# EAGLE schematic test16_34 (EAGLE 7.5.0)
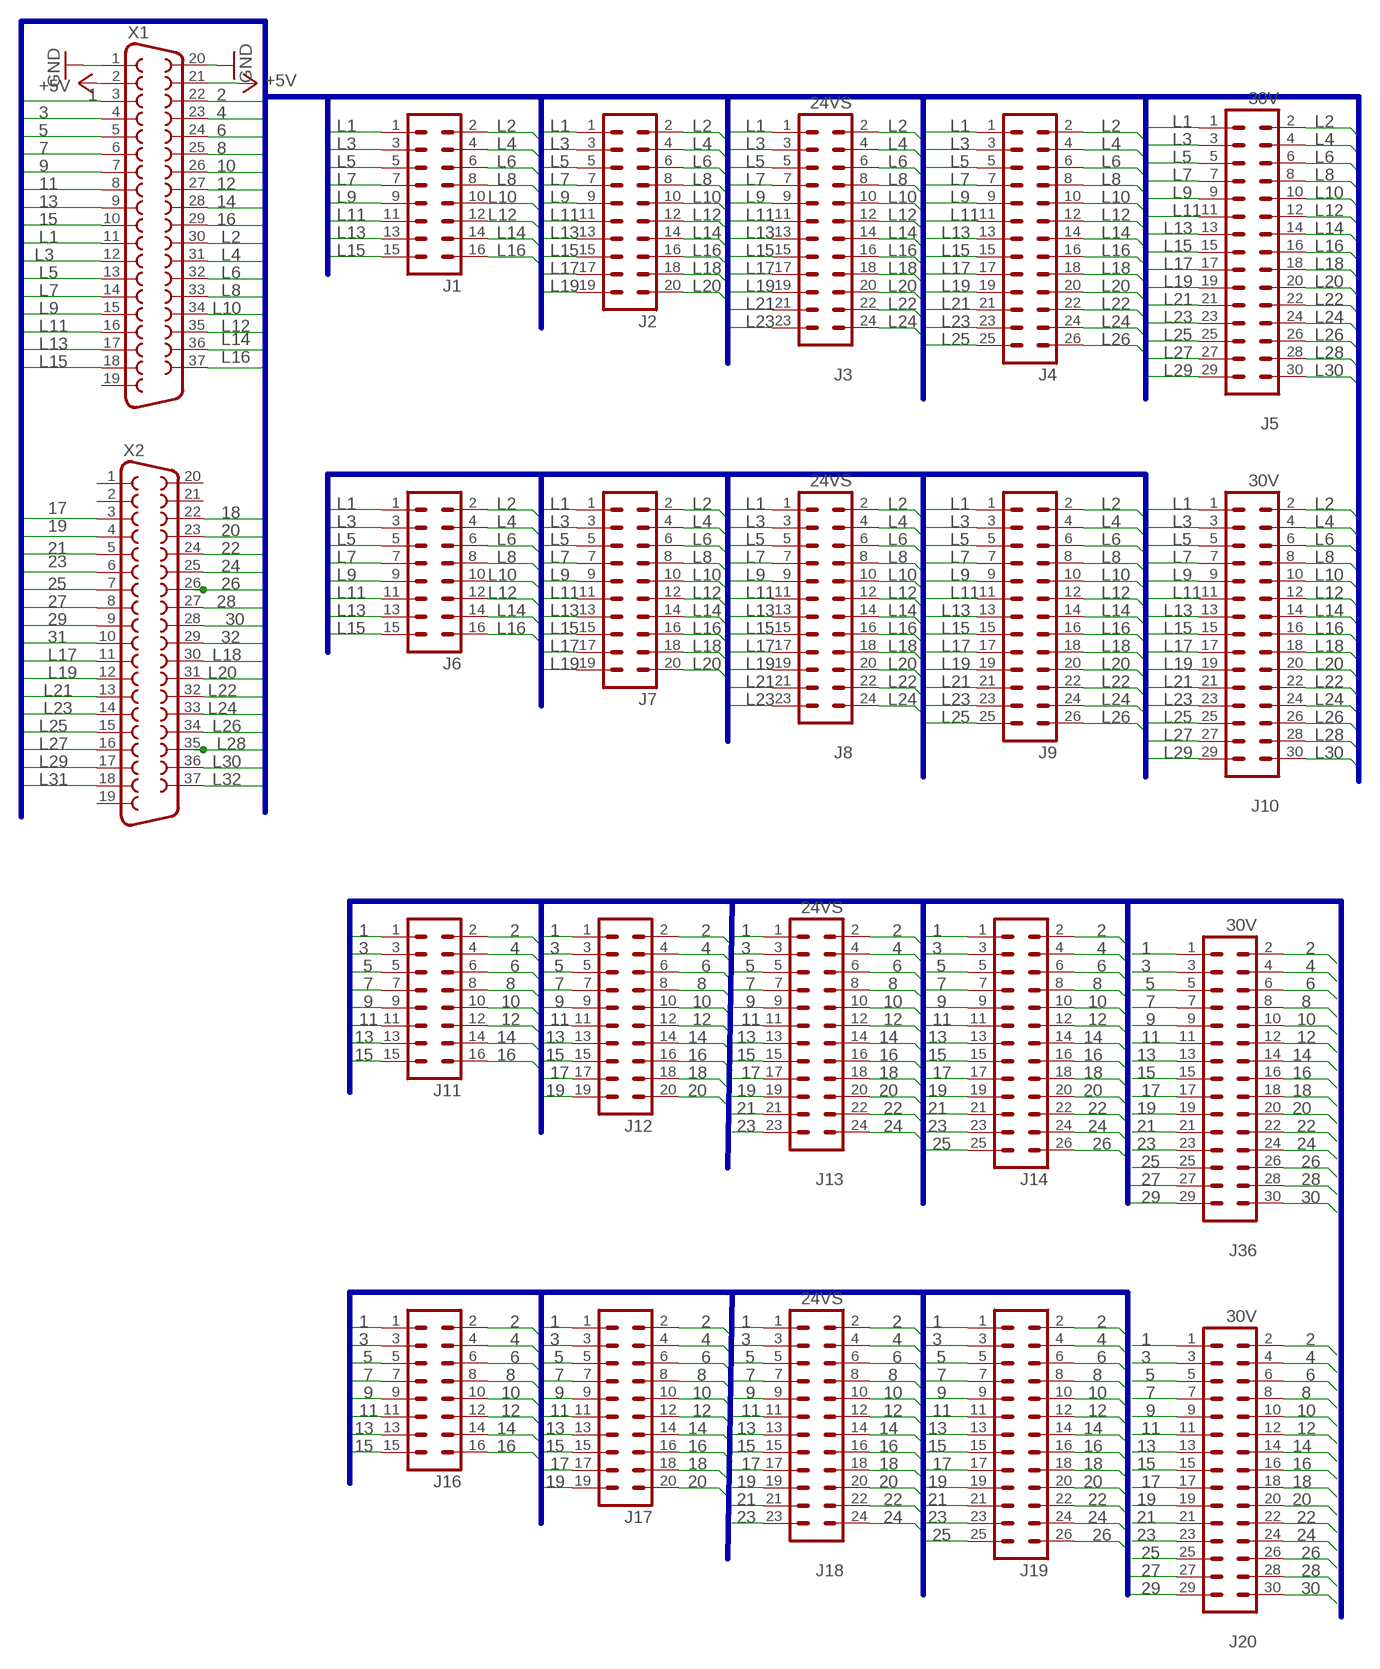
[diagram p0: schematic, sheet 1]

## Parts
J1  16V  [16V]
J2  20V  [20V]
J3  24VS  [24V]
J4  26V  [26V]
J5  30V  [30V]
J6  16V  [16V]
J7  20V  [20V]
J8  24VS  [24V]
J9  26V  [26V]
J10  30V  [30V]
J11  16V  [16V]
J12  20V  [20V]
J13  24VS  [24V]
J14  26V  [26V]
J16  16V  [16V]
J17  20V  [20V]
J18  24VS  [24V]
J19  26V  [26V]
J20  30V  [30V]
J36  30V  [30V]
X1  F37V  [F37V]
X2  F37V  [F37V]

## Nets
1: J11.1 J12.1 J13.1 J14.1 J16.1 J17.1 J18.1 J19.1 J20.1 J36.1 X1.3
2: J11.2 J12.2 J13.2 J14.2 J16.2 J17.2 J18.2 J19.2 J20.2 J36.2 X1.22
3: J11.3 J12.3 J13.3 J14.3 J16.3 J17.3 J18.3 J19.3 J20.3 J36.3 X1.4
4: J11.4 J12.4 J13.4 J14.4 J16.4 J17.4 J18.4 J19.4 J20.4 J36.4 X1.23
5: J11.5 J12.5 J13.5 J14.5 J16.5 J17.5 J18.5 J19.5 J20.5 J36.5 X1.5
6: J11.6 J12.6 J13.6 J14.6 J16.6 J17.6 J18.6 J19.6 J20.6 J36.6 X1.24
7: J11.7 J12.7 J13.7 J14.7 J16.7 J17.7 J18.7 J19.7 J20.7 J36.7 X1.6
8: J11.8 J12.8 J13.8 J14.8 J16.8 J17.8 J18.8 J19.8 J20.8 J36.8 X1.25
9: J11.9 J12.9 J13.9 J14.9 J16.9 J17.9 J18.9 J19.9 J20.9 J36.9 X1.7
10: J11.10 J12.10 J13.10 J14.10 J16.10 J17.10 J18.10 J19.10 J20.10 J36.10 X1.26
11: J11.11 J12.11 J13.11 J14.11 J16.11 J17.11 J18.11 J19.11 J20.11 J36.11 X1.8
12: J11.12 J12.12 J13.12 J14.12 J16.12 J17.12 J18.12 J19.12 J20.12 J36.12 X1.27
13: J11.13 J12.13 J13.13 J14.13 J16.13 J17.13 J18.13 J19.13 J20.13 J36.13 X1.9
14: J11.14 J12.14 J13.14 J14.14 J16.14 J17.14 J18.14 J19.14 J20.14 J36.14 X1.28
15: J11.15 J12.15 J13.15 J14.15 J16.15 J17.15 J18.15 J19.15 J20.15 J36.15 X1.10
16: J11.16 J12.16 J13.16 J14.16 J16.16 J17.16 J18.16 J19.16 J20.16 J36.16 X1.29
17: J12.17 J13.17 J14.17 J17.17 J18.17 J19.17 J20.17 J36.17 X2.3
18: J12.18 J13.18 J14.18 J17.18 J18.18 J19.18 J20.18 J36.18 X2.22
19: J12.19 J13.19 J14.19 J17.19 J18.19 J19.19 J20.19 J36.19 X2.4
20: J12.20 J13.20 J14.20 J17.20 J18.20 J19.20 J20.20 J36.20 X2.23
21: J13.21 J14.21 J18.21 J19.21 J20.21 J36.21 X2.5
22: J13.22 J14.22 J18.22 J19.22 J20.22 J36.22 X2.24
23: J13.23 J14.23 J18.23 J19.23 J20.23 J36.23 X2.6
24: J13.24 J14.24 J18.24 J19.24 J20.24 J36.24 X2.25
25: J14.25 J19.25 J20.25 J36.25 X2.7
26: J14.26 J19.26 J20.26 J36.26 X2.26
27: J20.27 J36.27 X2.8
28: J20.28 J36.28 X2.27
29: J20.29 J36.29 X2.9
30: J20.30 J36.30 X2.28
31: X2.10
32: X2.29
+5V: X1.2 X1.21
GND: X1.1 X1.20
L1: J1.1 J2.1 J3.1 J4.1 J5.1 J6.1 J7.1 J8.1 J9.1 J10.1 X1.11
L2: J1.2 J2.2 J3.2 J4.2 J5.2 J6.2 J7.2 J8.2 J9.2 J10.2 X1.30
L3: J1.3 J2.3 J3.3 J4.3 J5.3 J6.3 J7.3 J8.3 J9.3 J10.3 X1.12
L4: J1.4 J2.4 J3.4 J4.4 J5.4 J6.4 J7.4 J8.4 J9.4 J10.4 X1.31
L5: J1.5 J2.5 J3.5 J4.5 J5.5 J6.5 J7.5 J8.5 J9.5 J10.5 X1.13
L6: J1.6 J2.6 J3.6 J4.6 J5.6 J6.6 J7.6 J8.6 J9.6 J10.6 X1.32
L7: J1.7 J2.7 J3.7 J4.7 J5.7 J6.7 J7.7 J8.7 J9.7 J10.7 X1.14
L8: J1.8 J2.8 J3.8 J4.8 J5.8 J6.8 J7.8 J8.8 J9.8 J10.8 X1.33
L9: J1.9 J2.9 J3.9 J4.9 J5.9 J6.9 J7.9 J8.9 J9.9 J10.9 X1.15
L10: J1.10 J2.10 J3.10 J4.10 J5.10 J6.10 J7.10 J8.10 J9.10 J10.10 X1.34
L11: J1.11 J2.11 J3.11 J4.11 J5.11 J6.11 J7.11 J8.11 J9.11 J10.11 X1.16
L12: J1.12 J2.12 J3.12 J4.12 J5.12 J6.12 J7.12 J8.12 J9.12 J10.12 X1.35
L13: J1.13 J2.13 J3.13 J4.13 J5.13 J6.13 J7.13 J8.13 J9.13 J10.13 X1.17
L14: J1.14 J2.14 J3.14 J4.14 J5.14 J6.14 J7.14 J8.14 J9.14 J10.14 X1.36
L15: J1.15 J2.15 J3.15 J4.15 J5.15 J6.15 J7.15 J8.15 J9.15 J10.15 X1.18
L16: J1.16 J2.16 J3.16 J4.16 J5.16 J6.16 J7.16 J8.16 J9.16 J10.16 X1.37
L17: J2.17 J3.17 J4.17 J5.17 J7.17 J8.17 J9.17 J10.17 X2.11
L18: J2.18 J3.18 J4.18 J5.18 J7.18 J8.18 J9.18 J10.18 X2.30
L19: J2.19 J3.19 J4.19 J5.19 J7.19 J8.19 J9.19 J10.19 X2.12
L20: J2.20 J3.20 J4.20 J5.20 J7.20 J8.20 J9.20 J10.20 X2.31
L21: J3.21 J4.21 J5.21 J8.21 J9.21 J10.21 X2.13
L22: J3.22 J4.22 J5.22 J8.22 J9.22 J10.22 X2.32
L23: J3.23 J4.23 J5.23 J8.23 J9.23 J10.23 X2.14
L24: J3.24 J4.24 J5.24 J8.24 J9.24 J10.24 X2.33
L25: J4.25 J5.25 J9.25 J10.25 X2.15
L26: J4.26 J5.26 J9.26 J10.26 X2.34
L27: J5.27 J10.27 X2.16
L28: J5.28 J10.28 X2.35
L29: J5.29 J10.29 X2.17
L30: J5.30 J10.30 X2.36
L31: X2.18
L32: X2.37
Unconnected: X1.19 X2.1 X2.2 X2.19 X2.20 X2.21

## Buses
B$1

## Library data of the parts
J1 J6 J11 J16 = con-harting-v:16V: CONNECTOR; OC_FARNELL: unknown; OC_NEWARK: unknown
J2 J7 J12 J17 = con-harting-v:20V: CONNECTOR; OC_FARNELL: unknown; OC_NEWARK: unknown
J3 J8 J13 J18 = con-harting-v:24VS
J4 J9 J14 J19 = con-harting-v:26V: CONNECTOR; OC_FARNELL: unknown; OC_NEWARK: unknown
J5 J10 J20 J36 = con-harting-v:30V
X1 X2 = con-subd:F37: SUB-D; OC_FARNELL: unknown; OC_NEWARK: unknown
